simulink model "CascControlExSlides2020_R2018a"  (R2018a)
settings: Solver=ode4  StartTime=0.0  StopTime=100  FixedStep=0.001  RelTol=1e-3
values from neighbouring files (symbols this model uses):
  R = pidtune(P1*P2,R,omegab_des)    [CascadeControlSlides2020.m]
  R1 = pidtune(P1,R1,omegab_des)    [CascadeControlSlides2020.m]
  R2 = pidtune(P2,R2,10*omegab_des)    [CascadeControlSlides2020.m]

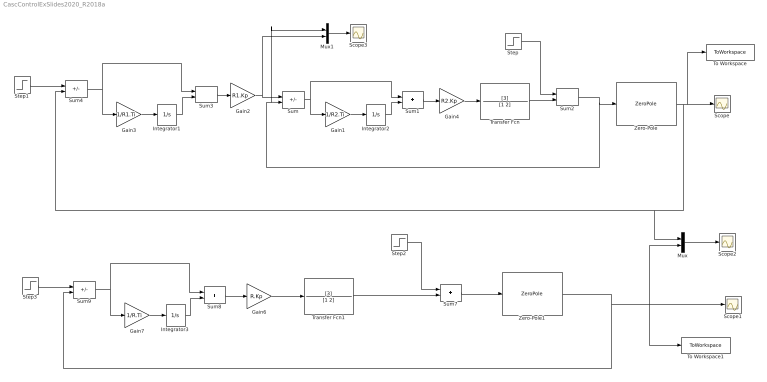
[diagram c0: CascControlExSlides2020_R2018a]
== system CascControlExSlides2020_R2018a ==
  Gain1 : Gain  Gain=1/R2.Ti
  Gain2 : Gain  Gain=R1.Kp
  Gain3 : Gain  Gain=1/R1.Ti
  Gain4 : Gain  Gain=R2.Kp
  Gain6 : Gain  Gain=R.Kp
  Gain7 : Gain  Gain=1/R.Ti
  Integrator1 : Integrator
  Integrator2 : Integrator
  Integrator3 : Integrator
  Mux : Mux  Inputs=2
  Mux1 : Mux  Inputs=2
  Scope{,1..3} (4 alike) : Scope
  Step : Step  Time=50  SampleTime=0
  Step1 : Step  Time=0  SampleTime=0
  Step2 : Step  Time=50  SampleTime=0
  Step3 : Step  Time=0  SampleTime=0
  Sum : Sum  Inputs=+-
  Sum{1..3,7..8} (5 alike) : Sum
  Sum4 : Sum  Inputs=+-
  Sum9 : Sum  Inputs=+-
  To Workspace : ToWorkspace  VariableName=ycasc  SaveFormat=Timeseries  SampleTime=-1
  To Workspace1 : ToWorkspace  VariableName=ysl  SaveFormat=Timeseries  SampleTime=-1
  Transfer Fcn : TransferFcn  Numerator=[3]  Denominator=[1 2]
  Transfer Fcn1 : TransferFcn  Numerator=[3]  Denominator=[1 2]
  Zero-Pole : ZeroPole  Zeros=[]  Poles=[-1 -1 -1]  Gain=10
  Zero-Pole1 : ZeroPole  Zeros=[]  Poles=[-1 -1 -1]  Gain=10
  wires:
  Gain4/1 -> Transfer Fcn/1
  Transfer Fcn/1 -> Sum2/2
  Sum2/1 -> Zero-Pole/1, Mux1/1, Sum/2
  Step/1 -> Sum2/1
  Integrator1/1 -> Sum3/2
  Sum3/1 -> Gain2/1
  Sum4/1 -> Sum3/1, Gain3/1
  Gain3/1 -> Integrator1/1
  Gain2/1 -> Mux1/2, Sum/1
  Zero-Pole/1 -> To Workspace/1, Scope/1, Sum4/2, Mux/1
  Step1/1 -> Sum4/1
  Step3/1 -> Sum9/1
  Zero-Pole1/1 -> To Workspace1/1, Mux/2, Scope1/1, Sum9/2
  Gain7/1 -> Integrator3/1
  Sum9/1 -> Gain7/1, Sum8/1
  Sum8/1 -> Gain6/1
  Integrator3/1 -> Sum8/2
  Step2/1 -> Sum7/1
  Sum7/1 -> Zero-Pole1/1
  Transfer Fcn1/1 -> Sum7/2
  Gain6/1 -> Transfer Fcn1/1
  Mux/1 -> Scope2/1
  Gain1/1 -> Integrator2/1
  Integrator2/1 -> Sum1/2
  Sum1/1 -> Gain4/1
  Sum/1 -> Gain1/1, Sum1/1
  Mux1/1 -> Scope3/1
